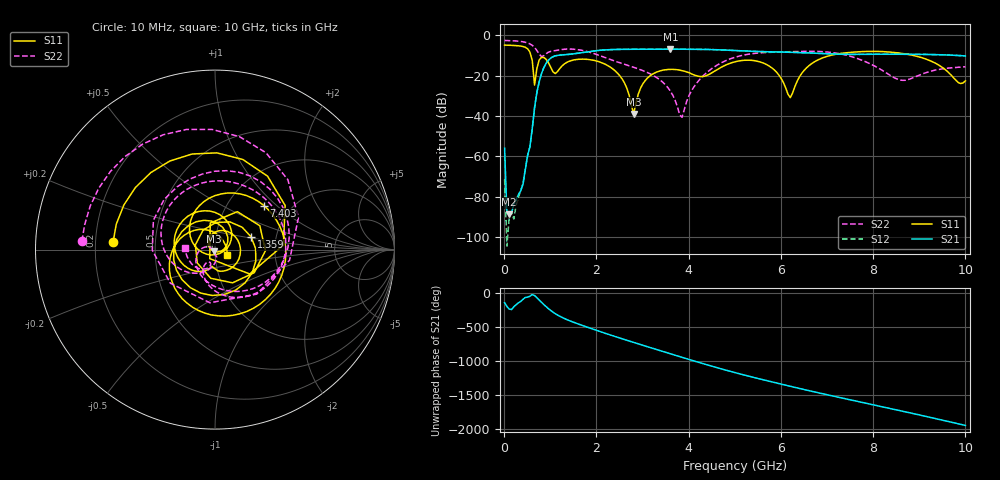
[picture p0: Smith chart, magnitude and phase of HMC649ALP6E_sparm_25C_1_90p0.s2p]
!Analog Devices Inc..
!GaAs MMIC 6-BIT DIGITAL PHASE SHIFTER, 3 - 6 GHz
!Filename: HMC649ALP6E_sparm_25C_1_90p0.s2p
!  :25C = 25degC
!  :_1_ = Sn1
!  :_90p0  = 90.0 state
!Device type:
!2 Port Calibration to sma connectors
!Phase Shifter:  0.000
!	Vss= -5V, Vdd= +5V , control Voltage = 0/ +5V
!Freq	S11	S11	S21	S21	S12	S12	S22	S22
! GHz	Mag dB	Degrees	Mag dB	Degrees	Mag dB	Degrees	Mag dB	Degrees
# GHZ S DB R 50.0
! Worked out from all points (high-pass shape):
!   201 points, 10 MHz to 10 GHz, reference 50 ohm
!   highest |S21| = -6.89 dB at 3.606 GHz (marker M1); lowest = -88.7 dB at 109.9 MHz (marker M2)
!   |S21| within 3 dB of the highest: 1.186 GHz to 9.722 GHz (8.536 GHz wide, 157 % of centre)
!   lowest |S11| = -39.0 dB at 2.807 GHz (marker M3), VSWR 1.02, Z = 49.5 - j0.996 ohm
!   |S11| at or under -10 dB: 579.1 MHz to 7.073 GHz (6.494 GHz wide, 170 % of centre); 8.869 GHz to end of sweep
!   |S22| runs from -40.7 to -2.6 dB; largest |S21 - S12| = 0.0013
!   S11 on the Smith chart (normalised r, x): 10 MHz: 0.27, +0.03; 1.359 GHz: 1.48, +0.22; 7.403 GHz: 1.47, +0.83; 10 GHz: 1.15, -0.06
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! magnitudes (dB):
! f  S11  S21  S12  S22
! 10 MHz  -4.9  -56.0  -71.4  -2.6
! 59.95 MHz  -4.9  -88.1  -104.5  -2.6
! 109.9 MHz  -5.0  -88.7  -90.2  -2.7
! 409.6 MHz  -5.6  -73.8  -73.1  -3.2
! 559.5 MHz  -8.4  -55.1  -55.2  -4.3
! 659.4 MHz  -24.7  -35.9  -35.9  -6.0
! 859.1 MHz  -11.0  -16.1  -16.1  -10.1
! 1.359 GHz  -13.4  -9.6  -9.5  -6.8
! 1.708 GHz  -11.8  -8.5  -8.5  -7.6
! 2.458 GHz  -18.8  -7.0  -7.0  -13.3
! 2.807 GHz  -39.0  -6.9  -6.9  -15.9
! 3.357 GHz  -17.8  -6.9  -6.9  -21.7
! 3.606 GHz  -16.9  -6.9  -6.9  -27.8
! 3.856 GHz  -17.5  -6.9  -6.9  -40.7
! 4.256 GHz  -20.5  -7.0  -7.0  -21.5
! 5.005 GHz  -13.1  -7.6  -7.6  -10.9
! 5.754 GHz  -15.4  -8.2  -8.2  -8.5
! 6.204 GHz  -30.9  -8.4  -8.4  -8.1
! 6.703 GHz  -13.5  -8.9  -8.9  -8.0
! 7.403 GHz  -8.7  -9.5  -9.5  -9.8
! 8.352 GHz  -8.3  -9.4  -9.4  -19.6
! 10 GHz  -22.6  -10.2  -10.2  -15.6
